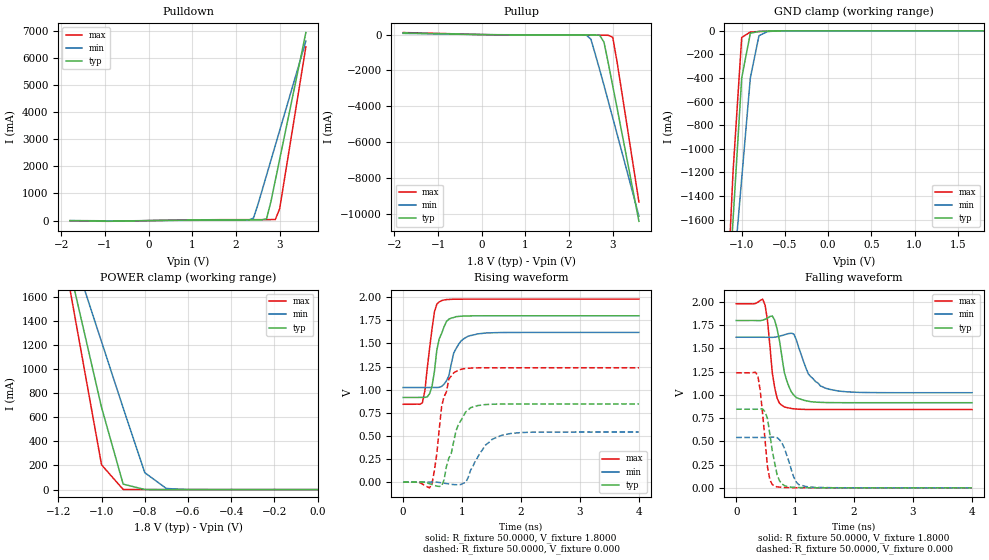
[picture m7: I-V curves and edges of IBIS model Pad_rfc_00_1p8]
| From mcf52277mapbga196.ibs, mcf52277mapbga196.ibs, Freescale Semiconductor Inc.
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|   Model Pad_rfc_00
[Model]   Pad_rfc_00_1p8
Model_type   3-state
Polarity   Non-Inverting
Enable   Active-High
Vmeas =   0.9000V
C_comp   1.7450pF   1.6200pF   1.8900pF
[Temperature Range]   25.0000   0.1500k   -40.0000
[Voltage Range]   1.8000V   1.6200V   1.9800V
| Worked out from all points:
|   slope of the pulldown table from 0 to 0.27 V, typ, clamps not added: 42 ohm
|   slope of the pullup table from 0 to 0.27 V, typ, clamps not added: 30.4 ohm
|   GND clamp passes 1 mA (typ) near -0.62 V on its own axis
|   POWER clamp passes 1 mA (typ) near -0.80 V on its own axis
|   rising waveform, R_fixture 50.0000, V_fixture 1.8000: 20-80 % time 157ps typ, 182ps min, 129ps max; typ from 0.916 V to 1.8 V
|   rising waveform, R_fixture 50.0000, V_fixture 0.000: 20-80 % time 254ps typ, 331ps min, 181ps max; typ from 0 V to 0.846 V
|   falling waveform, R_fixture 50.0000, V_fixture 1.8000: 20-80 % time 171ps typ, 282ps min, 118ps max; typ from 1.8 V to 0.916 V
|   falling waveform, R_fixture 50.0000, V_fixture 0.000: 20-80 % time 138ps typ, 168ps min, 111ps max; typ from 0.846 V to 0 V
[Pulldown]
| voltage   I(typ)   I(min)   I(max)
-1.8V     -1.93mA    -948uA     -3.57mA
-900mV    -18.6mA    -9.254mA   -24.67mA
2.3V      25.56mA    20.75mA    36.27mA
2.4V      25.68mA    96.64mA    36.43mA
2.5V      25.8mA     582.6mA    36.56mA
2.6V      26.8mA     1.131A     36.69mA
2.7V      71.34mA    1.68A      36.8mA
2.8V      707mA      2.228A     36.93mA
2.9V      1.486A     2.777A     40.84mA
3V        2.264A     3.325A     441.2mA
3.6V      6.936A     6.626A     6.415A
[Pullup]
| voltage   I(typ)   I(min)   I(max)
-1.8V     87.82mA    65.52mA    111.8mA
400mV     -11.94mA   -7.59mA    -17.89mA
2.4V      -19.35mA   -39.21mA   -28.48mA
2.5V      -21.05mA   -260.1mA   -28.69mA
2.7V      -39.08mA   -1.949A    -32.07mA
2.8V      -417.8mA   -2.828A    -35.46mA
2.9V      -1.62A     -3.734A    -40.57mA
3V        -2.851A    -4.641A    -149.6mA
3.1V      -4.098A    -5.547A    -1.532A
3.6V      -10.41A    -10.12A    -9.331A
[GND_clamp]
| voltage   I(typ)   I(min)   I(max)
-1.8V     -10.39A    -8.454A    -12.14A
-1.2V     -2.833A    -2.997A    -2.746A
-1.1V     -1.601A    -2.108A    -1.195A
-1V       -399mA     -1.252A    -56.61mA
-900mV    -20.31mA   -398.2mA   -10.19mA
-800mV    -5.193mA   -41.09mA   -5.939mA
-700mV    -2.389mA   -6.145mA   -2.797mA
-400mV    -10.19uA   -60.07uA   -3.537uA
1.8V      460.9pA    80.51nA    11.42pA
[POWER_clamp]
| voltage   I(typ)   I(min)   I(max)
-1.8V     6.91A      5.617A     8.169A
-1.2V     2.238A     2.322A     2.196A
-1.1V     1.459A     1.774A     1.2A
-1V       681mA      1.225A     205.3mA
-900mV    45.38mA    676.7mA    1.42mA
-800mV    926.3uA    140.3mA    9.915uA
-700mV    19.1uA     9.035mA    78.66nA
-600mV    427.3nA    583uA      682.7pA
0V        460.9pA    46.95nA    15.9pA
[Ramp]
| variable   typ   min   max
dV/dt_r   0.5074/0.2232n   0.3253/0.3248n   0.7425/0.1691n
dV/dt_f   0.5305/0.1630n   0.3580/0.2680n   0.6825/0.1106n
R_load = 50.0000
[Rising Waveform]
R_fixture = 50.0000
V_fixture = 1.8000
V_fixture_min = 1.6200
V_fixture_max = 1.9800
| time   V(typ)   V(min)   V(max)
0s        915.8mV    1.023V     842.4mV
326.5ps   917.2mV    1.023V     859.6mV
449ps     956.7mV    1.024V     1.451V
530.6ps   1.197V     1.024V     1.842V
571.4ps   1.431V     1.024V     1.926V
653.1ps   1.61V      1.036V     1.964V
775.5ps   1.764V     1.15V      1.977V
898ps     1.79V      1.445V     1.979V
1.143ns   1.799V     1.586V     1.98V
4ns       1.8V       1.62V      1.98V
[Rising Waveform]
R_fixture = 50.0000
V_fixture = 0.000
| time   V(typ)   V(min)   V(max)
0s        139.2pV    1.715nV    75.29pV
489.8ps   -25.99mV   984.8uV    -17.02mV
571.4ps   -43.7mV    -552.3uV   309.1mV
653.1ps   -42.61mV   -7.548mV   819.3mV
775.5ps   260.2mV    -19.95mV   1.117V
938.8ps   624.3mV    -28.28mV   1.213V
1.143ns   805.3mV    127.1mV    1.234V
1.388ns   838.8mV    396.1mV    1.237V
1.674ns   844.6mV    506.8mV    1.237V
4ns       845.7mV    542.2mV    1.237V
[Falling Waveform]
R_fixture = 50.0000
V_fixture = 1.8000
V_fixture_min = 1.6200
V_fixture_max = 1.9800
| time   V(typ)   V(min)   V(max)
0s        1.8V       1.62V      1.98V
449ps     1.804V     1.62V      2.03V
530.6ps   1.825V     1.62V      1.802V
612.2ps   1.849V     1.619V     1.239V
653.1ps   1.804V     1.621V     1.079V
816.3ps   1.242V     1.646V     870.9mV
1.02ns    971.3mV    1.591V     847.9mV
1.225ns   931.8mV    1.226V     843.3mV
1.51ns    917.8mV    1.073V     842.5mV
4ns       915.8mV    1.023V     842.4mV
[Falling Waveform]
R_fixture = 50.0000
V_fixture = 0.000
| time   V(typ)   V(min)   V(max)
0s        845.7mV    542.3mV    1.237V
367.3ps   846.4mV    542.3mV    1.204V
408.2ps   850.4mV    542.2mV    1.045V
530.6ps   745.8mV    542.2mV    227mV
571.4ps   577.3mV    543.6mV    84.64mV
653.1ps   266.8mV    547.1mV    18.05mV
775.5ps   42.56mV    483.9mV    4.905mV
1.02ns    4.188mV    61.42mV    708.4uV
1.184ns   1.701mV    13.93mV    157uV
4ns       997.1nV    10.62uV    1.242uV
